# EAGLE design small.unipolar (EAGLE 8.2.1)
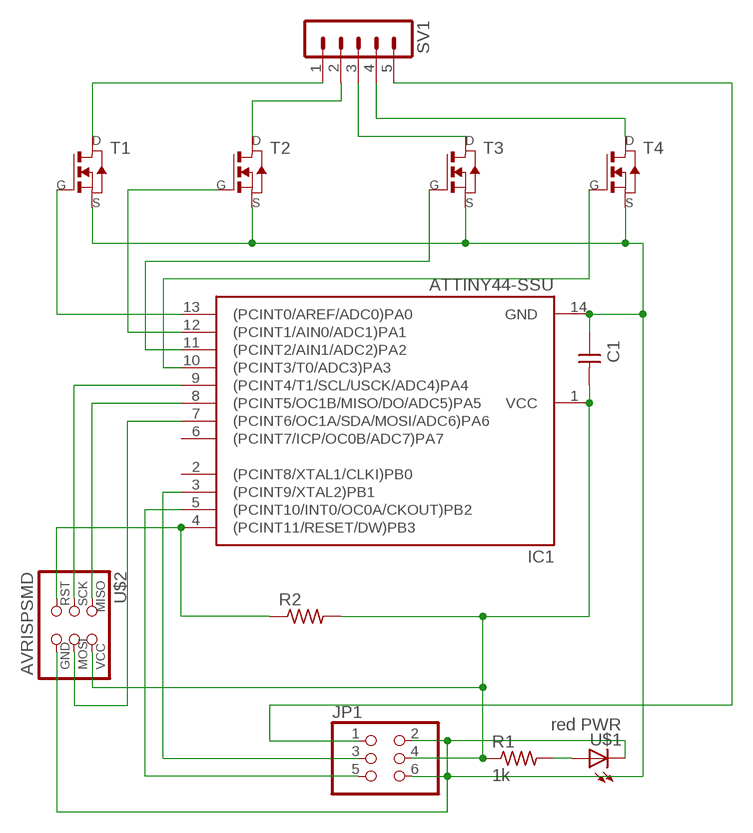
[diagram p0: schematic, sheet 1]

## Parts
C1  CAP-UNPOLARIZEDFAB  [C1206FAB]
IC1  ATTINY44-SSU  [SOIC14]
JP1  PINHD-2X3-SMD  [2X03SMD]
R1  1k  RES-US1206FAB  [R1206FAB]
R2  RES-US1206FAB  [R1206FAB]
SV1  MA05-1  [MA05-1]
T1  NMOSFETSOT23  [SOT-23]
T2  NMOSFETSOT23  [SOT-23]
T3  NMOSFETSOT23  [SOT-23]
T4  NMOSFETSOT23  [SOT-23]
U$1  red PWR  LEDFAB1206  [LED1206FAB]
U$2  AVRISPSMD  [2X03SMD]

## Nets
N$1: IC1.9((PCINT4/T1/SCL/USCK/ADC4)PA4) U$2.3(SCK)
N$2: R1.2 U$1.1(A)
N$3: JP1.1 SV1.5
N$4: IC1.5((PCINT10/INT0/OC0A/CKOUT)PB2) JP1.5
N$5: C1.1 IC1.14(GND) JP1.2 JP1.6 T1.2(S) T2.2(S) T3.2(S) T4.2(S) U$1.2(C) U$2.6(GND)
N$6: IC1.7((PCINT6/OC1A/SDA/MOSI/ADC6)PA6) U$2.4(MOSI)
N$7: IC1.13((PCINT0/AREF/ADC0)PA0) T1.3(G)
N$8: IC1.3((PCINT9/XTAL2)PB1) JP1.3
N$9: SV1.1 T1.1(D)
N$10: IC1.4((PCINT11/RESET/DW)PB3) R2.1 U$2.5(RST)
N$11: C1.2 IC1.1(VCC) JP1.4 R1.1 R2.2 U$2.2(VCC)
N$14: IC1.8((PCINT5/OC1B/MISO/DO/ADC5)PA5) U$2.1(MISO)
N$15: SV1.2 T2.1(D)
N$16: SV1.3 T3.1(D)
N$17: SV1.4 T4.1(D)
N$23: IC1.10((PCINT3/T0/ADC3)PA3) T4.3(G)
N$24: IC1.11((PCINT2/AIN1/ADC2)PA2) T3.3(G)
N$25: IC1.12((PCINT1/AIN0/ADC1)PA1) T2.3(G)
Unconnected: IC1.2((PCINT8/XTAL1/CLKI)PB0) IC1.6((PCINT7/ICP/OC0B/ADC7)PA7)

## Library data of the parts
C1 = fab:CAP-UNPOLARIZED
IC1 = fab:ATTINY44
JP1 = fab:PINHD-2X3-SMD: PIN HEADER
R1 R2 = fab:RES-US: Resistor (US Symbol)
SV1 = con-lstb:MA05-1: PIN HEADER; OC_FARNELL: unknown; OC_NEWARK: unknown
T1-T4 = fab:NMOSFET: MOS FET
U$1 = fab:LED: LED
U$2 = fab:AVRISP

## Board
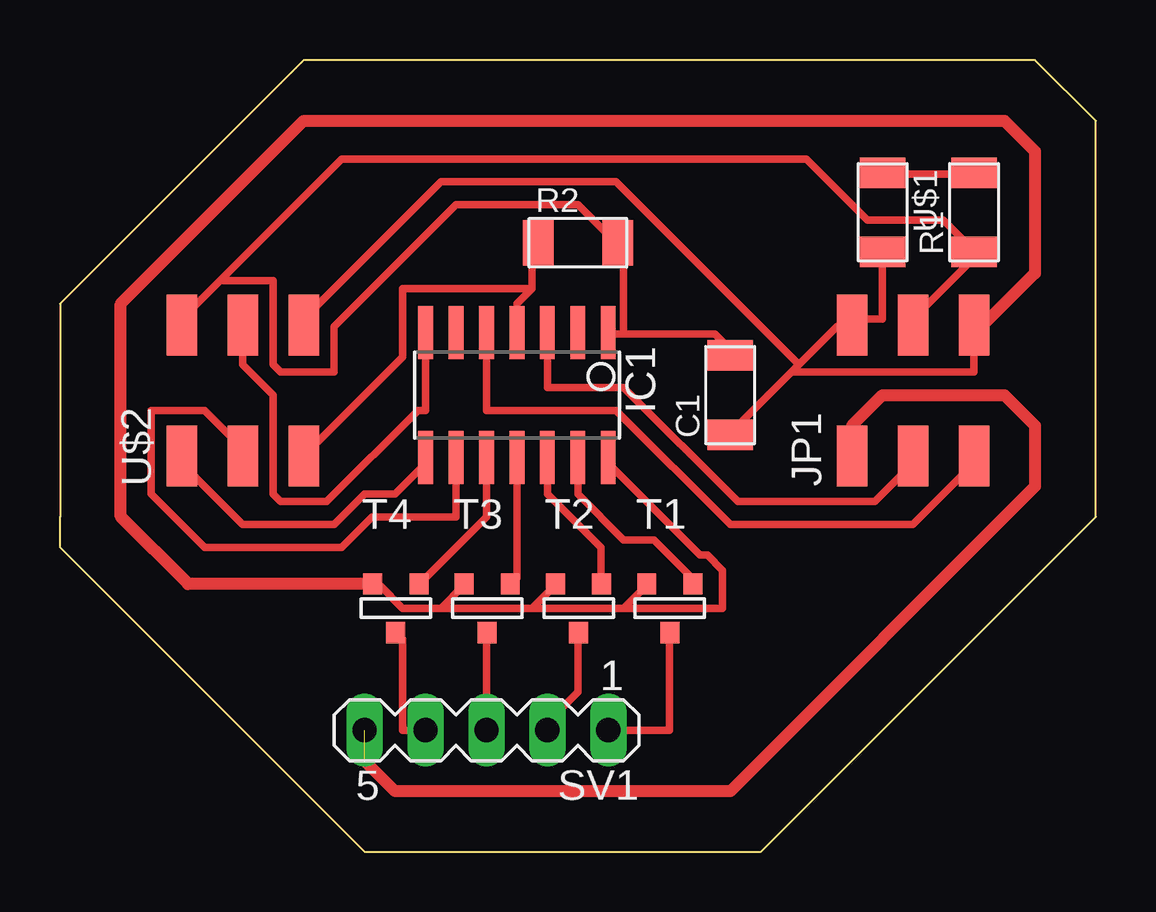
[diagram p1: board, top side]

Size 43.18 x 33.02 mm. Coordinates in mm from the lower left corner, seen from the top.
Outline: 10.16,33.02 0,22.86 0,13.97 0,12.7 12.7,0 29.21,0 43.18,13.97 43.18,30.48 40.64,33.02 10.16,33.02
Copper layers (1*16): Top 0.035mm / dielectric 1.5mm / Bottom 0.035mm
Design rules "default *": minimum track width 12mil, minimum drill 0.35mm, track to track 16mil, track to pad 16mil, pad to pad 16mil, via to via 16mil, smd to smd 16mil, copper to edge 40mil, drill to drill 6mil, minimum pad ring 10mil, minimum via ring 8mil, stop-mask expansion 4mil, vias tented up to drill 0mil, thermal gap 10mil

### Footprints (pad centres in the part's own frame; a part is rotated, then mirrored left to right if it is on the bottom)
C1206FAB = smd 1.27 x 1.905: 1 -1.651,0; 2 1.651,0
SOIC14 = smd 0.61 x 2.21: 1 -3.81,-2.603; 2 -2.54,-2.603; 3 -1.27,-2.603; 4 0,-2.603; 5 1.27,-2.603; 6 2.54,-2.603; 7 3.81,-2.603; 8 3.81,2.603; 9 2.54,2.603; 10 1.27,2.603; 11 0,2.603; 12 -1.27,2.603; 13 -2.54,2.603; 14 -3.81,2.603
2X03SMD = smd 2.54 x 1.27: 1 -2.54,2.54; 2 2.92,2.54; 3 -2.54,0; 4 2.92,0; 5 -2.54,-2.54; 6 2.92,-2.54
R1206FAB = smd 1.27 x 1.905: 1 -1.651,0; 2 1.651,0
MA05-1 = drill 1.016 long: 1 -5.08,0; 2 -2.54,0; 3 0,0; 4 2.54,0; 5 5.08,0
SOT-23 = smd 0.787 x 0.889: 1 0.025,-1.016; 2 -0.94,1.016; 3 0.991,1.016
LED1206FAB = smd 1.27 x 1.905: 1 -1.651,0; 2 1.651,0

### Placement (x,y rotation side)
C1  27.94,19.05 90 top
IC1  19.05,19.05 180 top
JP1  35.56,19.05 90 top
R1  38.1,26.67 90 top
R2  21.59,25.4 0 top
SV1  17.78,5.08 180 top
T1  25.4,10.16 0 top
T2  21.59,10.16 0 top
T3  17.78,10.16 0 top
T4  13.97,10.16 0 top
U$1  34.29,26.67 270 top
U$2  7.62,19.05 90 top

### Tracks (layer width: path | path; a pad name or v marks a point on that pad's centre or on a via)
N$1
  Top 0.305: IC1.9 16.51,13.97 13.02,13.97 11.75,12.7 6.03,12.7 3.81,14.92 3.81,18.41 6.03,18.41 7.62,16.83 U$2.3
N$2
  Top 0.305: U$1.1 34.29,28.26 38.1,28.26 R1.2
N$3  (1 unrouted)
  Top 0.508: JP1.1 33.02,17.78 34.29,19.05 39.37,19.05 40.64,17.78 40.64,15.24 27.94,2.54 13.97,2.54 12.7,3.81
N$4
  Top 0.305: IC1.5 17.78,18.41 23.18,18.41 27.94,13.65 35.56,13.65 38.1,16.19 JP1.5
N$5
  Top 0.305: 15.88,10.16 14.29,10.16 13.34,11.11 T4.2 | 15.88,10.16 16.83,11.11 T3.2 | 19.68,10.16 20.64,11.11 T2.2 | 15.88,10.16 19.68,10.16 | 23.5,10.16 24.45,11.11 T1.2 | 19.68,10.16 23.5,10.16 | 23.5,10.16 27.62,10.16 27.62,11.75 26.99,12.38 26.67,12.38 22.86,16.19 IC1.14 | 30.8,20.32 32.38,21.91 33.02,21.91 JP1.2 33.02,22.23 34.29,22.23 U$1.2 | 30.8,20.32 30.48,20 | 30.48,20 27.94,17.46 C1.1 | 30.8,20.32 23.18,27.94 15.88,27.94 10.16,22.23 U$2.6 | JP1.6 38.1,21.59 38.1,20 30.48,20
  Top 0.508: T4.2 5.33,11.18 2.54,13.97 2.54,22.86 10.16,30.48 39.37,30.48 40.64,29.21 40.64,24.13 38.1,21.59
N$6
  Top 0.305: IC1.7 15.24,18.41 14.92,18.41 11.11,14.61 9.21,14.61 8.89,14.92 8.89,19.05 7.62,20.32 U$2.4
N$7
  Top 0.305: IC1.13 21.59,14.92 23.5,13.02 24.77,13.02 26.35,11.43 T1.3
N$8
  Top 0.305: IC1.3 20.32,19.37 23.5,19.37 28.26,14.61 33.97,14.61 35.56,16.19 JP1.3
N$9
  Top 0.305: SV1.1 25.4,5.08 25.4,8.89 T1.1
N$10
  Top 0.305: 19.68,23.5 19.68,25.4 R2.1 | 19.68,23.5 19.05,22.86 IC1.4 | U$2.5 14.29,20.64 14.29,23.5 19.68,23.5
N$11
  Top 0.305: 23.5,21.59 22.86,21.59 IC1.1 | 23.5,21.59 27.3,21.59 27.94,20.95 C1.2 | 23.5,21.59 23.5,25.4 R2.2 23.18,25.4 21.59,26.99 16.51,26.99 11.43,21.91 11.43,20 9.21,20 8.89,20.32 8.89,23.81 6.67,23.81 | JP1.4 35.56,22.23 38.1,24.77 R1.1 38.1,25.08 36.83,26.35 33.65,26.35 31.11,28.89 11.75,28.89 6.67,23.81 | 6.67,23.81 5.08,22.23 U$2.2
N$14
  Top 0.305: U$2.1 5.08,16.19 7.62,13.65 11.43,13.65 12.7,14.92 13.97,14.92 15.24,16.19 IC1.8
N$15
  Top 0.305: SV1.2 20.32,5.4 21.59,6.67 21.59,8.89 T2.1
N$16
  Top 0.305: SV1.3 17.78,8.89 T3.1
N$17
  Top 0.305: SV1.4 14.29,5.08 14.29,8.89 T4.1
N$23
  Top 0.305: IC1.10 17.78,13.97 15.24,11.43 T4.3
N$24
  Top 0.305: IC1.11 19.05,11.43 T3.3
N$25
  Top 0.305: IC1.12 20.32,14.92 22.54,12.7 22.54,11.43 T2.3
